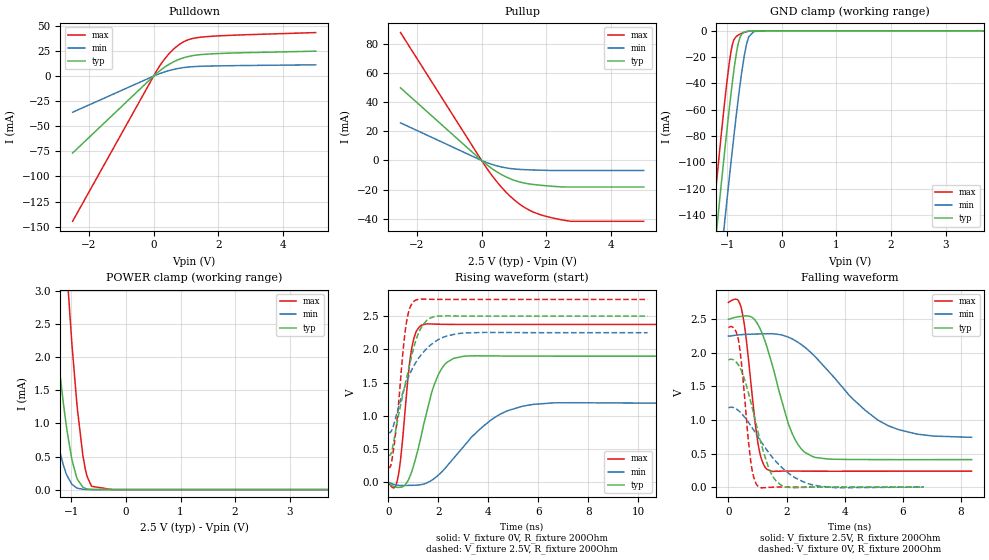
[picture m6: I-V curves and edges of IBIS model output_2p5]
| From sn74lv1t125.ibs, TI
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|   output_2p5 Model
[Model]   output_2p5
Model_type   3-state
Polarity   Non-Inverting
Vmeas = 1.25
Vref = 0
Cref = 50pF
Rref = 250
|   typ   min   max
|   (nom PVT)   (fast PVT)   (slow PVT)
C_comp   3.305e-12   3.211e-12   3.402e-12
| Where nom  PVT is Nominal Process, 2.5V, 40C
|   Fast PVT is Strong Process,  2.75V, -40C
|   Slow PVT is Weak Process,   2.25V, 140C
[Voltage Range]   2.5   2.25   2.75
|Junction Temperature
[Temperature Range]   40   140   -40
[Pullup Reference]   2.5   2.25   2.75
[Pulldown Reference]   0   0   0
[Power Clamp Reference]   2.5   2.25   2.75
[GND Clamp Reference]   0   0   0
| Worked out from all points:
|   slope of the pulldown table from 0 to 0.375 V, typ, clamps not added: 38.7 ohm
|   slope of the pullup table from 0 to 0.375 V, typ, clamps not added: 58.2 ohm
|   GND clamp passes 1 mA (typ) near -0.68 V on its own axis
|   POWER clamp passes 1 mA (typ) near -1.10 V on its own axis
|   falling waveform, V_fixture 2.5V, R_fixture 200Ohm: 20-80 % time 838ps typ, 2.04ns min, 387ps max; typ from 2.5 V to 0.41 V
|   rising waveform, V_fixture 0V, R_fixture 200Ohm: 20-80 % time 783ps typ, 1.82ns min, 363ps max; typ from 0 V to 1.9 V
|   rising waveform, V_fixture 2.5V, R_fixture 200Ohm: 20-80 % time 741ps typ, 1.04ns min, 374ps max; typ from 0.41 V to 2.5 V
|   falling waveform, V_fixture 0V, R_fixture 200Ohm: 20-80 % time 697ps typ, 1.26ns min, 309ps max; typ from 1.9 V to 0 V
[Pulldown]
|   Voltage   I(typ)   I(min)   I(max)
-2.5V     -76.69mA   -36.03mA   -144.7mA
87.5mV    2.582mA    1.203mA    5.003mA
351.8mV   9.211mA    4.304mA    17.62mA
500mV     12.21mA    5.707mA    23.21mA
756mV     16.27mA    7.587mA    30.67mA
951.3mV   18.5mA     8.584mA    34.6mA
1.125V    19.9mA     9.179mA    36.81mA
1.548V    21.66mA    9.862mA    39.08mA
5V        24.83mA    11.22mA    43.36mA
[GND Clamp]
|   Voltage   I(typ)   I(min)   I(max)
-2.5V     -719.7mA   -763.9mA   -692.1mA
-1.35V    -216.9mA   -270mA     -180.4mA
-1.114V   -118.7mA   -172.6mA   -80.84mA
-1.065V   -98.78mA   -152.6mA   -61.13mA
-1.026V   -83.62mA   -137.3mA   -46.46mA
-962.7mV  -59.56mA   -112.5mA   -24.67mA
-899.5mV  -37.2mA    -88.35mA   -9.599mA
-802.5mV  -10.48mA   -53.46mA   -3.396mA
-740.5mV  -2.875mA   -33.5mA    -1.977mA
-624.5mV  -398.4uA   -7.069mA   -460uA
-511mV    -63.18uA   -492.1uA   -56.18uA
5V        0A         0A         0A
[Pullup]
|   Voltage   I(typ)   I(min)   I(max)
-2.5V     49.98mA    25.88mA    88.05mA
141.5mV   -2.625mA   -1.3mA     -4.754mA
351.8mV   -6.101mA   -2.934mA   -11.26mA
635mV     -9.98mA    -4.59mA    -18.96mA
890.8mV   -12.69mA   -5.569mA   -24.82mA
1.135V    -14.58mA   -6.098mA   -29.45mA
1.438V    -16.05mA   -6.427mA   -33.82mA
1.758V    -16.93mA   -6.661mA   -36.92mA
2.192V    -17.78mA   -6.908mA   -39.58mA
2.747V    -18.27mA   -6.915mA   -41.87mA
5V        -18.27mA   -6.915mA   -41.88mA
[POWER Clamp]
|   Voltage   I(typ)   I(min)   I(max)
-2.5V     19.18mA    10.25mA    35.65mA
-1.65V    6.189mA    2.895mA    13.59mA
-1.496V   4.419mA    1.933mA    10.34mA
-1.351V   2.953mA    1.158mA    7.55mA
-1.21V    1.764mA    570.2uA    5.168mA
-1.083V   906.5uA    216.2uA    3.319mA
-993mV    466.5uA    84.08uA    2.236mA
-905mV    188.9uA    26.85uA    1.353mA
-787.5mV  35.64uA    4.874uA    507.4uA
-712.5mV  10.21uA    1.583uA    199.6uA
-630mV    2.454uA    455.5nA    49.99uA
5V        0A         0A         0A
[Ramp]
R_load = 200
|   typ   min   max
dV/dt_r   1.13845/7.79891e-10   0.711374/1.81658e-09   1.42459/3.62901e-10
dV/dt_f   1.25396/8.37107e-10   0.902739/2.02212e-09   1.50796/3.87053e-10
[Falling Waveform]
V_fixture = 2.5V
V_fixture_min = 2.25V
V_fixture_max = 2.75V
R_fixture = 200Ohm
|   Time   V(typ)   V(min)   V(max)
0s        2.5V       2.25V      2.75V
300ps     2.533V     2.264V     2.793V
450ps     2.543V     2.27V      2.651V
600ps     2.549V     2.274V     2.248V
1.025ns   2.413V     2.28V      633.7mV
1.325ns   2.088V     2.284V     265.5mV
2.075ns   930.3mV    2.23V      239.1mV
2.675ns   506.7mV    2.067V     237.2mV
5.5ns     408.9mV    914.6mV    236.6mV
8.375ns   409.5mV    740.6mV    236.7mV
[Rising Waveform]
V_fixture = 0V
V_fixture_min = 0V
V_fixture_max = 0V
R_fixture = 200Ohm
|   Time   V(typ)   V(min)   V(max)
0s        542.1pV    8.118nV    750.4pV
350ps     -73.34mV   -41.07mV   17.5mV
500ps     -71.38mV   -45.51mV   386.2mV
900ps     125.3mV    -43.76mV   1.932V
1.325ns   719.3mV    -31.83mV   2.363V
1.975ns   1.599V     102mV      2.378V
2.6ns     1.863V     358.6mV    2.375V
4.075ns   1.902V     929.1mV    2.374V
5.375ns   1.898V     1.146V     2.374V
13.68ns   1.897V     1.186V     2.374V
[Rising Waveform]
V_fixture = 2.5V
V_fixture_min = 2.25V
V_fixture_max = 2.75V
R_fixture = 200Ohm
|   Time   V(typ)   V(min)   V(max)
0s        410.1mV    745.4mV    236.7mV
100ps     429mV      760.9mV    257.7mV
250ps     690.9mV    911.5mV    616.2mV
600ps     1.353V     1.374V     2.023V
725ps     1.563V     1.509V     2.407V
875ps     1.812V     1.645V     2.639V
1.1ns     2.136V     1.804V     2.74V
1.65ns    2.466V     2.052V     2.752V
2.725ns   2.501V     2.233V     2.75V
10.38ns   2.5V       2.25V      2.75V
[Falling Waveform]
V_fixture = 0V
V_fixture_min = 0V
V_fixture_max = 0V
R_fixture = 200Ohm
|   Time   V(typ)   V(min)   V(max)
0s        1.897V     1.186V     2.374V
225ps     1.879V     1.175V     2.347V
350ps     1.814V     1.138V     2.176V
450ps     1.729V     1.096V     1.84V
775ps     1.258V     910.3mV    366.3mV
1ns       858.8mV    760.9mV    21.12mV
1.45ns    222mV      476.5mV    -2.806mV
1.95ns    2.77mV     247.7mV    1.167mV
3.075ns   1.002mV    18.27mV    -87.82uV
6.725ns   -82.85uV   924uV      -1.378uV
